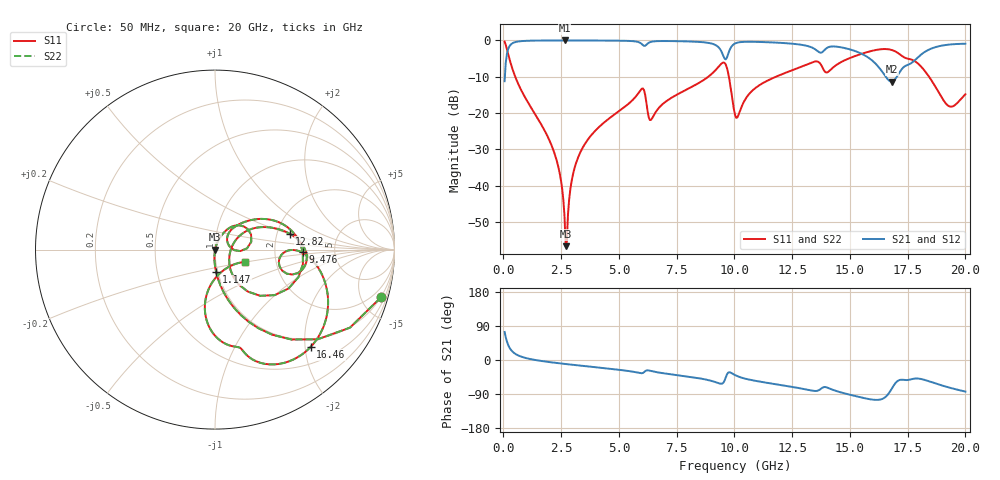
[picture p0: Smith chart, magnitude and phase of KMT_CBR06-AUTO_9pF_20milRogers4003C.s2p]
! Data measured by Modelithics Inc. support@modelithics.com 813-866-6335
! KEMET CBR06-AUTO 9pF, Pad Width= 0.851mm, Pad Length= 0.64mm, Pad Gap= 0.62mm, 20mil Rogers 4003C substrate Data, January 2022
# hz S ma R 50
! 2 Port Network Data from SP1.SP block
! freq  magS11  angS11  magS21  angS21  magS12  angS12  magS22  angS22
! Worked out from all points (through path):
!   401 points, 50 MHz to 20 GHz, reference 50 ohm
!   highest |S21| = -0.01 dB at 2.643 GHz (marker M1); lowest = -11.4 dB at 16.81 GHz (marker M2)
!   group delay of S21, straight-line fit = 13.2 ps
!   lowest |S11| = -56.7 dB at 2.693 GHz (marker M3), VSWR 1.00, Z = 50.1 - j0.128 ohm
!   |S11| at or under -10 dB: 509.1 MHz to 8.87 GHz (8.36 GHz wide, 178 % of centre); 9.759 GHz to 11.8 GHz (2.042 GHz wide, 18.9 % of centre); 18.42 GHz to end of sweep
!   |S22| runs from -56.7 to -0.3 dB; largest |S21 - S12| = 0
!   S11 on the Smith chart (normalised r, x): 50 MHz: 0.98, -6.94; 1.147 GHz: 0.98, -0.25; 9.476 GHz: 2.91, -0.12; 12.82 GHz: 2.34, +0.51; 16.46 GHz: 0.83, -2.12; 20 GHz: 1.39, -0.19
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5e7  0.9617 -16.1  0.2739 73.9  0.2739 73.9  0.9617 -16.1
3.99125e8  0.3955 -68.2  0.9178 21.7  0.9178 21.7  0.3955 -68.2
1.14725e9  0.1258 -87.0  0.9913 2.7  0.9913 2.7  0.1258 -87.0
2.2445e9  0.02565 -95.5  0.9987 -7.4  0.9987 -7.4  0.02565 -95.5
2.6435e9  0.003774 -86.2  0.999 -10.3  0.999 -10.3  0.003774 -86.2
2.693375e9  0.001458 -61.3  0.999 -10.6  0.999 -10.6  0.001458 -61.3
3.0425e9  0.01574 73.4  0.9988 -13.0  0.9988 -13.0  0.01574 73.4
3.391625e9  0.03148 72.8  0.9983 -15.2  0.9983 -15.2  0.03148 72.8
5.985125e9  0.2155 31.6  0.8943 -35.0  0.8943 -35.0  0.2155 31.6
6.384125e9  0.08001 28.6  0.9547 -29.0  0.9547 -29.0  0.08001 28.6
6.73325e9  0.118 50.1  0.9791 -33.2  0.9791 -33.2  0.118 50.1
9.476375e9  0.4897 -1.8  0.6622 -62.1  0.6622 -62.1  0.4897 -1.8
1.0025e10  0.09388 -32.7  0.9064 -39.6  0.9064 -39.6  0.09388 -32.7
1.2818e10  0.4249 12.0  0.8785 -74.4  0.8785 -74.4  0.4249 12.0
1.336662e10  0.4992 0.7  0.7957 -80.8  0.7957 -80.8  0.4992 0.7
1.491275e10  0.557 -7.3  0.7654 -90.3  0.7654 -90.3  0.557 -7.3
1.645888e10  0.7602 -45.4  0.3485 -101.0  0.3485 -101.0  0.7602 -45.4
1.670825e10  0.7513 -54.8  0.2773 -85.7  0.2773 -85.7  0.7513 -54.8
1.6808e10  0.7387 -58.8  0.2697 -76.0  0.2697 -76.0  0.7387 -58.8
1.825438e10  0.3753 -98.0  0.6984 -52.9  0.6984 -52.9  0.3753 -98.0
1.925188e10  0.1261 -70.0  0.8733 -71.9  0.8733 -71.9  0.1261 -70.0
2e10  0.1812 -21.8  0.9002 -83.3  0.9002 -83.3  0.1812 -21.8
